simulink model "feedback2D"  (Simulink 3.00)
settings: Solver=ode45  StartTime=0.0  StopTime=50  MaxStep=.01  RelTol=1e-3  AbsTol=1e-3

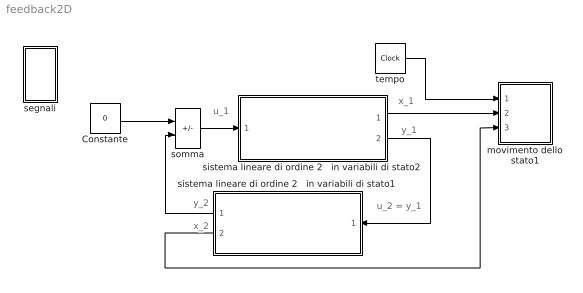
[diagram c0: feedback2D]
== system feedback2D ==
  note: x_1
  note: x_2
  note: u_2 = y_1
  note: y_1
  note: y_2
  note: u_1
  Constante : Constant  Value=0
  movimento dello stato1 : Subsystem  mask(grafico 3D){xlim=[0,20], ylim=[-2 3], zlim=[-2,2], view=[10 30]}
      mask prompts: xlim "t [min,max]:"; ylim "x1 [min,max]:"; zlim "x2 [min,max]:"; view "Orientamento:"
      mask help: Movimento dello stato del sistema Introdurre gli intervalli di rappresentazione del tempo e dello stato
      mask init:
      | st=-1;
  segnali : Subsystem
  sistema lineare di ordine 2   in variabili di stato1 : Subsystem  Orientation=left  mask(2D state-space system ){F=-1, G=1, H=1, x0_c=0}
      mask prompts: F "dynamic matrix A2:"; G "input matrix B2:"; H "output matrix C2:"; x0_c "initial condition:"
  sistema lineare di ordine 2   in variabili di stato2 : Subsystem  mask(2D state-space system ){A=-1, B=1, C=1, x0_s=3}
      mask prompts: A "dynamic matrix A1:"; B "input matrix B1:"; C "output matrix C1:"; x0_s "initial condition:"
  somma : Sum  Inputs=+-  SaturateOnIntegerOverflow=on
  tempo : Clock
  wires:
  tempo/1 -> movimento dello stato1/1(x)
  sistema lineare di ordine 2   in variabili di stato2/1(x) -> movimento dello stato1/2(y)
  somma/1 -> sistema lineare di ordine 2   in variabili di stato2/1(in_1)
  Constante/1 -> somma/1
  sistema lineare di ordine 2   in variabili di stato2/2(y) -> sistema lineare di ordine 2   in variabili di stato1/1(in_1)
  sistema lineare di ordine 2   in variabili di stato1/1(y) -> somma/2
  sistema lineare di ordine 2   in variabili di stato1/2(x) -> movimento dello stato1/3(z)

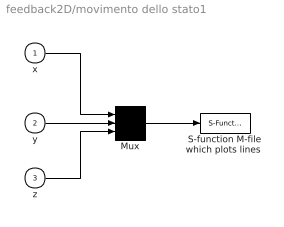
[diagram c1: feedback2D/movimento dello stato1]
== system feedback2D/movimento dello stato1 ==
  x : Inport  Port=1  PortWidth=-1  SampleTime=-1  DataType=auto
  y : Inport  Port=2  PortWidth=-1  SampleTime=-1  DataType=auto
  z : Inport  Port=3  PortWidth=-1  SampleTime=-1  DataType=auto
  Mux : Mux  Inputs=3
  "S-function M-file which plots lines " : S-Function  FunctionName=sfunxyz  Parameters=xlim,ylim,zlim,view,st  PortCounts=[]  SFunctionModules=''
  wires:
  z/1 -> Mux/3
  y/1 -> Mux/2
  x/1 -> Mux/1
  Mux/1 -> "S-function M-file which plots lines "/1

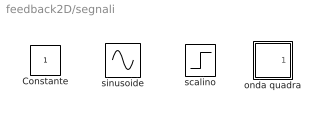
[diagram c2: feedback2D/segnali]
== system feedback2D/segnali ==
  Constante : Constant  Value=1
  onda quadra : Subsystem  mask(Pulse Generator){}
      mask help: Pulse Generator.
      mask init:
      | Ts=@1; du=@2; ht=@3; stt=@4; ini=ones(length(ht),1); st1=rem(stt,Ts); st2=rem(stt+du,Ts);if(Ts<=1.2*du),ini=zeros(length(ht),1);end;
  scalino : Step  Time=0  Before=0  After=1  SampleTime=-1
  sinusoide : Sin  Amplitude=1  Frequency=1  Phase=0  SampleTime=-1

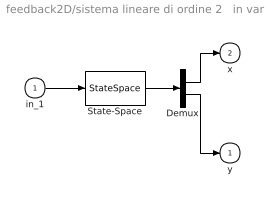
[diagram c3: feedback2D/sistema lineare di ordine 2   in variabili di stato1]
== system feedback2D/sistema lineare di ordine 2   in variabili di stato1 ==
  in_1 : Inport  Port=1  PortWidth=-1  SampleTime=-1  DataType=auto
  Demux : Demux  Outputs=2
  State-Space : StateSpace  A=F  B=G  C=[1 H]'  D=[0 0]'  X0=x0_c
  y : Outport  Port=1
  x : Outport  Port=2
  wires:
  in_1/1 -> State-Space/1
  State-Space/1 -> Demux/1
  Demux/1 -> x/1
  Demux/2 -> y/1

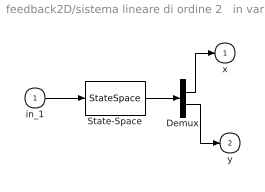
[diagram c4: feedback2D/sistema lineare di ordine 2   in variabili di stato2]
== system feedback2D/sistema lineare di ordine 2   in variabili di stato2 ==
  in_1 : Inport  Port=1  PortWidth=-1  SampleTime=-1  DataType=auto
  Demux : Demux  Outputs=2
  State-Space : StateSpace  A=A  B=B  C=[1 C]'  D=[0 0]'  X0=x0_s
  x : Outport  Port=1
  y : Outport  Port=2
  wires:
  in_1/1 -> State-Space/1
  State-Space/1 -> Demux/1
  Demux/1 -> x/1
  Demux/2 -> y/1

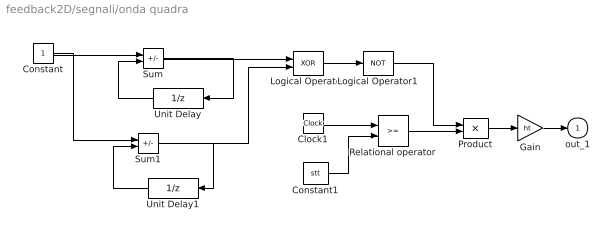
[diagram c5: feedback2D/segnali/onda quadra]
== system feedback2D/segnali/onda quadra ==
  Clock1 : Clock
  Constant : Constant  Value=1
  Constant1 : Constant  Value=stt
  Gain : Gain  Gain=ht  SaturateOnIntegerOverflow=on
  Logical Operator : Logic  Operator=XOR  Inputs=2
  Logical Operator1 : Logic  Operator=NOT  Inputs=1
  Product : Product  Inputs=2  SaturateOnIntegerOverflow=on
  Relational operator : RelationalOperator  Operator=>=
  Sum : Sum  Inputs=+-  SaturateOnIntegerOverflow=on
  Sum1 : Sum  Inputs=+-  SaturateOnIntegerOverflow=on
  Unit Delay : UnitDelay  Orientation=left  X0=0  SampleTime=[Ts,st1]
  Unit Delay1 : UnitDelay  Orientation=left  X0=ini  SampleTime=[Ts,st2]
  out_1 : Outport  Port=1
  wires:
  Logical Operator1/1 -> Product/1
  Logical Operator/1 -> Logical Operator1/1
  Constant1/1 -> Relational operator/2
  Gain/1 -> out_1/1
  Product/1 -> Gain/1
  Relational operator/1 -> Product/2
  Clock1/1 -> Relational operator/1
  Unit Delay/1 -> Sum/2
  Unit Delay1/1 -> Sum1/2
  Constant/1 -> Sum/1, Sum1/1
  Sum/1 -> Unit Delay/1, Logical Operator/1
  Sum1/1 -> Unit Delay1/1, Logical Operator/2
